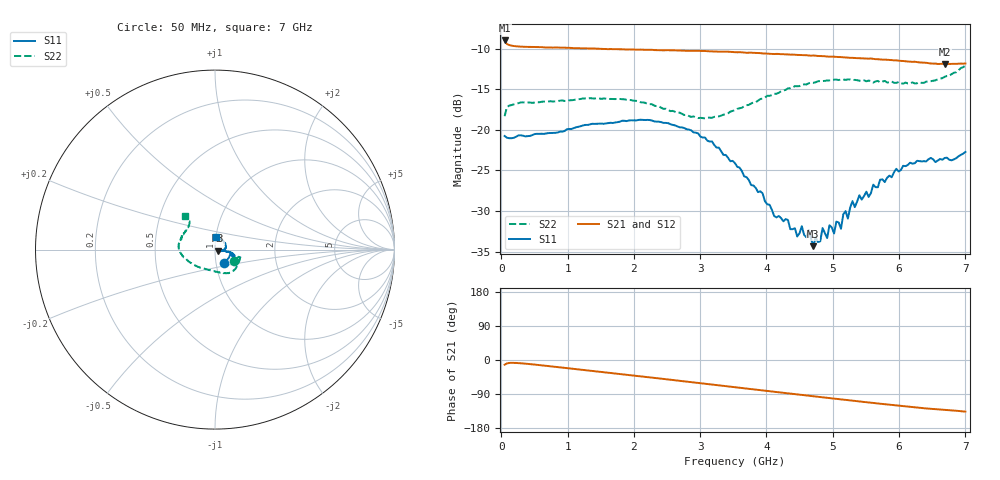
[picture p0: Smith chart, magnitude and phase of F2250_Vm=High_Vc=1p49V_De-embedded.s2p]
! Integrated Device Technology
! Corporate Headquarters
! 6024 Silver Creek Valley Road
! San Jose, CA 95138  USA
! Phone:  1-408-284-8200
! Toll Free:  1-800-223-1366
! Webpage:  http://www.idt.com/
! Timing and RF Division
! 515 Groton Road, Suite 102
! Westford, MA 01886-6024
! Device:  F2250
! Description: Voltage Variable RF Attenuator
! Frequency:  50.0 -  6000.00 MHz
! Package:  3x3 mm Thin QFN Plastic Package: 16 pin
! Ports:  2 RF, 3 DC
!  Pin  1  = GND
!  Pin  2  = NC
!  Pin  3  = RF1  = Port 1
!  Pin  4  = NC
!  Pin  5  = GND
!  Pin  6  = GND
!  Pin  7  = GND
!  Pin  8  = GND
!  Pin  9  = NC
!  Pin 10  = RF2  = Port 2
!  Pin 11  = NC
!  Pin 12  = GND
!  Pin 13  = GND
!  Pin 14  = VCNTRL
!  Pin 15  = VDD
!  Pin 16  = VMODE
! Vcntrl:  1.490 Volts
! Vmode:  +3.300 Volts
! Vdd:  +3.30  Volts
! Current:  1.330 mA
! Data:  The device was measured on a the F2250 evaluation board which has
!  individual transmission lines to the RF pins.  Data was collected
!  using a calibrated network analyzer.  The evaluation board was
!  de-embedded using a TRL calibration technique.
!  The reference plane is the edge of the package pin.
! Misc:  SN 10
!  Action Tracker AT0258
! Date Measured:  2014-11-26
! Date:  2015-10-15  MJV
! Note:
!  Integrated Device Technology supplies this data as a sample of measured
!  data at the package pin for this product.  Your particular data for this
!  product may vary.
!  Data was taken at 25 degrees C.
!  Integrated Device Technology reserves the right to change this data at anytime.
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# GHz S dB R 50
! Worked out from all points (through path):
!   201 points, 50 MHz to 7 GHz, reference 50 ohm
!   highest |S21| = -8.97 dB at 50 MHz (marker M1); lowest = -11.9 dB at 6.687 GHz (marker M2)
!   group delay of S21, straight-line fit = 54.3 ps
!   lowest |S11| = -34.3 dB at 4.707 GHz (marker M3), VSWR 1.04, Z = 51.9 - j0.623 ohm
!   |S11| at or under -10 dB: start of sweep to end of sweep
!   |S22| runs from -18.6 to -12.1 dB; largest |S21 - S12| = 0.0014
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0.05  -20.75 -55.7  -8.97 -12.5  -8.97 -12.4  -18.31 -31.1
0.29325  -20.66 -12.5  -9.74 -8.6  -9.73 -8.6  -16.62 -14.5
1.2315  -19.45 -20.8  -9.95 -26.2  -9.94 -26.2  -16.12 -42.1
2.37825  -18.99 -16.4  -10.17 -48.6  -10.19 -48.6  -17.08 -70.0
2.969  -20.43 -10.9  -10.24 -60.5  -10.26 -60.6  -18.54 -97.8
3.525  -24.10 -8.4  -10.43 -71.8  -10.43 -71.9  -17.57 -132.6
4.11575  -30.61 -9.0  -10.65 -83.8  -10.62 -83.9  -15.56 -159.5
4.32425  -31.11 -12.8  -10.70 -88.0  -10.71 -88.0  -14.88 -166.3
4.46325  -33.14 -14.5  -10.75 -90.8  -10.78 -90.8  -14.61 -169.8
4.637  -32.33 -14.8  -10.83 -94.3  -10.83 -94.3  -14.26 -175.1
4.7065  -34.33 -18.2  -10.83 -95.7  -10.84 -95.7  -14.19 -176.1
4.81075  -33.73 -24.1  -10.90 -97.7  -10.90 -97.7  -13.98 -178.2
4.8455  -32.10 -21.0  -10.92 -98.4  -10.91 -98.4  -13.97 -179.0
4.915  -33.33 -19.3  -10.96 -99.8  -10.95 -99.8  -13.91 178.9
4.94975  -31.76 -19.2  -10.97 -100.5  -10.96 -100.5  -13.90 178.2
5.1235  -32.18 -17.7  -11.03 -103.9  -11.02 -104.0  -13.80 173.9
5.15825  -30.41 -20.3  -11.05 -104.6  -11.05 -104.6  -13.79 173.5
5.22775  -30.93 -12.0  -11.09 -105.9  -11.09 -106.0  -13.78 171.7
5.29725  -28.77 -9.7  -11.12 -107.3  -11.11 -107.3  -13.87 170.3
5.85325  -25.64 0.2  -11.37 -118.0  -11.38 -118.1  -14.13 155.0
6.68725  -23.46 46.4  -11.89 -131.6  -11.87 -131.8  -13.45 132.0
7  -22.71 84.4  -11.82 -136.1  -11.84 -136.2  -12.07 131.9
